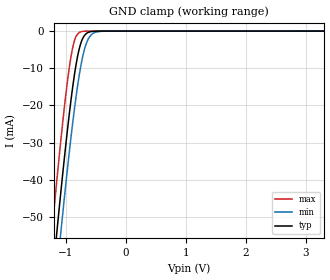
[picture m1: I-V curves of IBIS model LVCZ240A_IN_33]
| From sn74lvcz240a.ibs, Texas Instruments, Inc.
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[Model]   LVCZ240A_IN_33
Model_type  Input
Vinl = 0.8
Vinh = 2
| variable   typ   min   max
C_comp   3.5pF   NA   NA
[Temperature Range]   40   100   -40
| Ambient temperature   25   85   -40
[Voltage range]   3.3   3   3.6
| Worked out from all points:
|   GND clamp passes 1 mA (typ) near -0.68 V on its own axis
[GND Clamp]
| LVCZ240A_IN_33
|   Voltage   I(typ)   I(min)   I(max)
-5.5V     -872.3mA   -880mA     -863mA
-1.235V   -68.47mA   -79.32mA   -54.53mA
-1.155V   -55.02mA   -65.9mA    -41.02mA
-1.13V    -50.91mA   -61.78mA   -36.92mA
-1.085V   -43.65mA   -54.48mA   -29.72mA
-960mV    -24.78mA   -35.18mA   -11.94mA
-865mV    -12.71mA   -22.05mA   -3.093mA
-790mV    -5.74mA    -13.27mA   -568.9uA
-715mV    -1.873mA   -6.62mA    -78.61uA
-645mV    -520uA     -2.804mA   -11.73uA
-565mV    -106.8uA   -850.2uA   -1.322uA
3.3V      1.114nA    59.61nA    6.193pA
